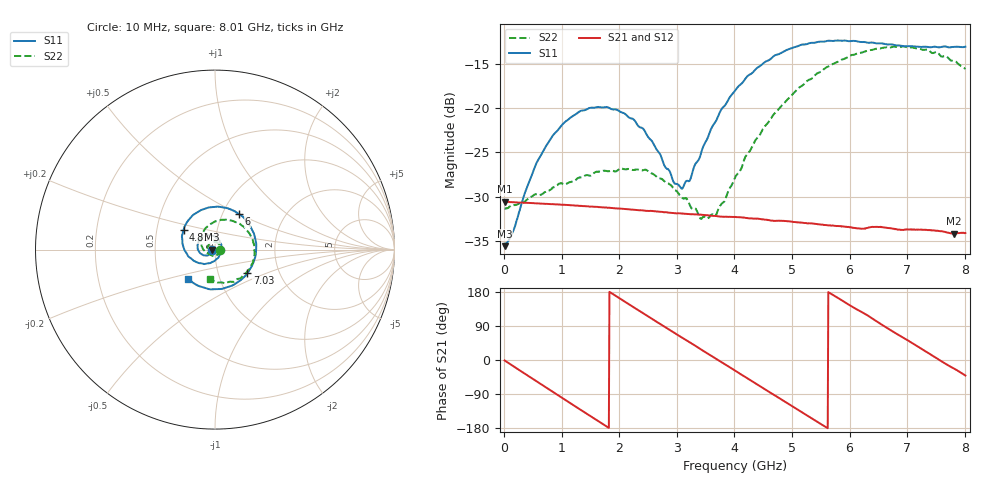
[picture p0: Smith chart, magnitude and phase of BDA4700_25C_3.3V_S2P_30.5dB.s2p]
!Agilent Technologies,E5071B,MY42404982,A.09.10
!Date: Mon Oct 20 18:15:54 2025
!Data & Calibration Information:
!Freq	S11:SOLT2(ON)	S21:SOLT2(ON)	S12:SOLT2(ON)	S22:SOLT2(ON)
# Hz S RI R 50
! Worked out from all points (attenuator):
!   801 points, 10 MHz to 8.01 GHz, reference 50 ohm
!   highest |S21| = -30.54 dB at 20 MHz (marker M1); lowest = -34.1 dB at 7.81 GHz (marker M2)
!   lowest |S11| = -35.6 dB at 10 MHz (marker M3), VSWR 1.03, Z = 48.4 - j0.101 ohm
!   |S11| at or under -10 dB: start of sweep to end of sweep
!   |S22| runs from -32.5 to -13.0 dB; largest |S21 - S12| = 0.00037
!   S11 on the Smith chart (normalised r, x): 10 MHz: 0.97, -0.00; 4.83 GHz: 0.69, +0.16; 6 GHz: 1.19, +0.50; 7.03 GHz: 1.38, -0.38; 8.01 GHz: 0.71, -0.24
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1e7  -0.0166 -0.00105  0.0297 -0.000653  0.0297 -0.000676  0.0272 -0.000814
2e7  -0.017 -0.00168  0.0297 -0.00107  0.0297 -0.00118  0.0271 -0.00108
7e8  -0.0485 -0.0332  0.01 -0.0271  0.0101 -0.0271  0.00615 -0.033
1.03e9  -0.0786 -0.0232  -0.006 -0.0279  -0.00597 -0.0279  -0.0163 -0.0335
1.35e9  -0.0968 0.00574  -0.0193 -0.0204  -0.0193 -0.0204  -0.0364 -0.0183
2.08e9  -0.0521 0.078  -0.0246 0.0111  -0.0247 0.0112  -0.0303 0.0337
2.68e9  0.0235 0.0517  -0.00363 0.0258  -0.00367 0.0259  0.0127 0.0383
2.95e9  0.0356 0.0132  0.00777 0.0244  0.00774 0.0243  0.0255 0.0241
3.1e9  0.0337 -0.0108  0.0135 0.0216  0.0133 0.0216  0.0287 0.012
3.23e9  0.0261 -0.0296  0.0176 0.0182  0.0175 0.0181  0.028 0.003
3.54e9  -0.0121 -0.0675  0.0239 0.00707  0.0239 0.007  0.0142 -0.0194
3.69e9  -0.0393 -0.0764  0.0246 0.001  0.0246 0.000934  0.0017 -0.0252
4.01e9  -0.1049 -0.0687  0.0216 -0.0114  0.0215 -0.0113  -0.031 -0.0259
4.36e9  -0.1639 -0.0127  0.0115 -0.0209  0.0116 -0.0209  -0.0656 0.00118
4.83e9  -0.1755 0.1087  -0.00622 -0.0223  -0.00602 -0.0224  -0.0764 0.0706
5.35e9  -0.0738 0.2214  -0.0202 -0.00952  -0.0201 -0.00964  -0.0157 0.1466
6e9  0.1333 0.198  -0.0173 0.0123  -0.0175 0.0123  0.1306 0.1467
6.68e9  0.2283 -0.0133  0.00306 0.0209  0.00312 0.0209  0.219 0.000653
7.03e9  0.1803 -0.1324  0.0133 0.0158  0.0134 0.0158  0.1989 -0.0929
7.45e9  0.0485 -0.2163  0.0201 0.00371  0.0201 0.00368  0.1134 -0.1702
7.81e9  -0.0862 -0.2044  0.0182 -0.00744  0.0182 -0.00748  0.0181 -0.1838
8.01e9  -0.1491 -0.1649  0.0149 -0.0129  0.015 -0.0129  -0.0296 -0.1635
